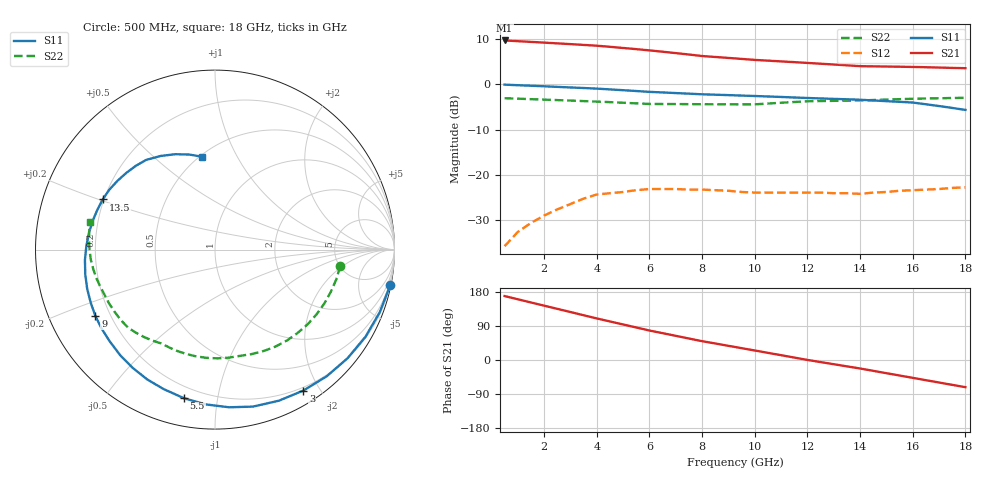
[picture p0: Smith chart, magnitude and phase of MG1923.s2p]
! MGF1923  (Ta=25deg. C, VDS=3V, lDS=10mA)
! From 1996/1997 GaAs FET/MMIC Data book
# GHZ S MA R 50
!  Freq.  S11  S21  S12  S22
!  GHz  (mag)  (ang)  (mag)  (ang)  (mag)  (ang)  (mag)  (ang)
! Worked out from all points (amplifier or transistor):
!   36 points, 500 MHz to 18 GHz, reference 50 ohm
!   highest |S21| = 9.8 dB at 500 MHz (marker M1)
!   |S21| within 3 dB of that: start of sweep to 7.302 GHz
!   unconditionally stable (mu >= 1): 9.746 GHz to end of sweep
!   at 3.5 GHz: K = 0.34, MSG = 17.1 dB, |S12| = -25.4 dB
!   at 9.5 GHz: K = 0.97, MSG = 14.8 dB, |S12| = -23.9 dB
!   at 18 GHz: K = 1.35, MAG = 9.7 dB, |S12| = -22.9 dB
!   lowest NFmin = 0.68 dB at 2 GHz
!   S11 on the Smith chart (normalised r, x): 500 MHz: 0.20, -9.93; 3 GHz: 0.16, -1.80; 5.5 GHz: 0.14, -0.80; 9 GHz: 0.14, -0.25; 13.5 GHz: 0.20, +0.21; 18 GHz: 0.51, +0.73
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0.5  0.996 -11.5  3.084 168.7  0.016 81.0  0.704 -7.4
1  0.982 -20.8  3.028 160.3  0.023 74.8  0.696 -13.7
2  0.955 -39.3  2.918 143.4  0.035 62.5  0.679 -26.3
2.5  0.941 -48.6  2.863 135.0  0.041 56.4  0.671 -32.6
3  0.927 -57.9  2.808 126.6  0.047 50.2  0.663 -38.9
3.5  0.914 -67.1  2.752 118.1  0.054 44.1  0.654 -45.2
4  0.9 -76.4  2.697 109.7  0.06 37.9  0.646 -51.5
4.5  0.882 -84.9  2.621 101.7  0.062 32.6  0.637 -57.9
5  0.864 -93.4  2.545 93.8  0.064 27.4  0.627 -64.2
5.5  0.846 -101.8  2.469 85.8  0.067 22.1  0.617 -70.6
6  0.828 -110.3  2.393 77.8  0.069 16.8  0.608 -76.9
6.5  0.816 -117.5  2.312 70.8  0.069 12.8  0.607 -82.8
7.5  0.791 -131.8  2.152 56.7  0.068 4.8  0.605 -94.6
8  0.778 -139.0  2.071 49.7  0.068 0.8  0.604 -100.5
9  0.762 -151.0  1.973 37.4  0.066 -3.2  0.603 -110.1
9.5  0.753 -156.9  1.924 31.3  0.064 -5.1  0.602 -114.8
11  0.727 -175.4  1.805 12.7  0.063 -9.8  0.627 -128.9
12.5  0.7 166.8  1.701 -5.5  0.063 -13.1  0.655 -143.1
13.5  0.685 155.9  1.633 -16.8  0.062 -14.3  0.662 -153.0
15.5  0.642 133.3  1.575 -40.9  0.066 -22.7  0.687 -171.0
16.5  0.603 120.1  1.555 -53.3  0.068 -29.7  0.699 -179.6
18  0.522 97.8  1.517 -71.7  0.072 -42.7  0.712 167.7
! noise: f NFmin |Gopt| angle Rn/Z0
2  0.68  0.82  18.5  0.47
4  0.75  0.695  36  0.42
8  1.3  0.573  81.2  0.38
12  1.8  0.489  115.8  0.34
18  2.55  0.362  173  0.42
